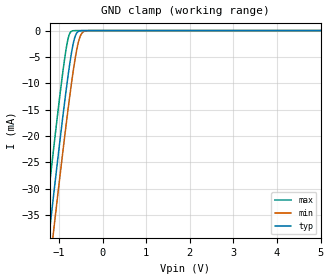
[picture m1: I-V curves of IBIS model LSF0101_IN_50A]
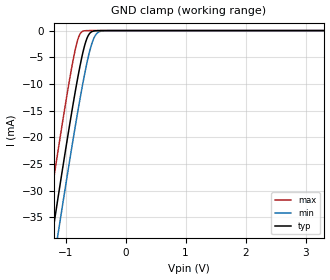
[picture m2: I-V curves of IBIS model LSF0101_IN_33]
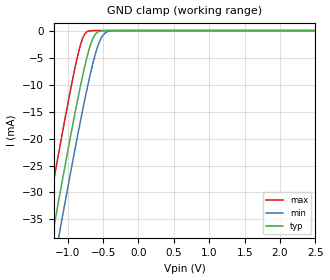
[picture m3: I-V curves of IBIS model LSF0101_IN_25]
|Texas Instruments Incorporated
| Single Bidirectional Multi-Voltage Level Translator
| for Open-Drain & Push-Pull Application
| Marketing part#   Digital Voltage Range   Package-type   #pins
| LSF0102DCT   1.2V-5.5V   SSOP   8
| LSF0102DCU   1.2V-5.5V   VSSOP   8
| This device can be powered at the following Vccs:
|  5 volt Vcc
|  3.3 volt Vcc
|  2.5 volt Vcc
|  1.8 volt Vcc
|  1.2 volt Vcc
[IBIS Ver]   4.1
[File name]   lsf0102.ibs
[File Rev]   1.0
[Date]   08/01/2014
[Source]
| Texas Instruments Incorporated.
| 12500 TI Blvd
| Dallas, TX -75243
[Notes]   Revision History:
| Rev 1.0: 8/01/2014
| - Initial version of the model
| - Model generated from simulations in TISPICE
| - C_comp although listed in numerical order of value are
|   obtained from varying PVT conditions. For PVT conditions for
|   each specific value refer the buffer description under
|   respective [Model]. IBIS model user is responsible for using
|   appropriate C_comp to simulate for Signal Integrity.
| - Non-monotonic data due to FET characteristics.
| - POWER clamp data deleted as there is no power-clmp diode.
[Disclaimer]
| This model is designed as an aid for customers of Texas Instruments.
| TI and its licensors and suppliers make no warranties, either expressed
| or implied, with respect to this  model, including the warranties of
| merchantability or fitness for a particular purpose. The model is
| provided solely on an "as is" basis. The entire risk as to its quality
| and performance is with the customer.
| This file provides unique models under the [Model Selector] for each Vcc.
| For operation at a specific Vcc, select the appropriate model after each
| [Model Selector] keyword.
[Copyright]
 (C) Copyright 2014 Texas Instruments Incorporated.All rights reserved.
|   Device
[Component]   LSF0102DCT
[Manufacturer]   TI
[Package]   |SSOP, 8 pin DCT
|   typ   min   max
R_pkg   0.0495   0.0439   0.0557
L_pkg   2.0203n   1.8892n   2.1572n
C_pkg   0.0923p   0.0784p   0.1044p
[Pin]  signal_name   model_name   R_pin   L_pin   C_pin
1   GND   GND   0.05353   2.1389n   0.1044p
2   VREF_A   LSF0101_IO   0.04507   1.9025n   0.0813p
3   A1   LSF0101_IO   0.04637   1.9443n   0.0839p
4   A2   LSF0101_IO   0.05217   2.0711n   0.1026p
5   B2   LSF0101_IO   0.05569   2.1572n   0.1042p
6   B1   LSF0101_IO   0.04687   1.9375n   0.0793p
7   VREF_B   LSF0101_IO   0.04389   1.8892n   0.0784p
8   EN   LSF0101_IN   0.05272   2.1213n   0.1042p
[Series Switch Groups]
| Function Group States
On  1 /   | A1 -> B1 EN HIGH
Off 1 /   | EN LOW
[Series Pin Mapping]   pin_2   model_name   function_table_group
3   6   LSF0101_IO_S   1
4   5   LSF0101_IO_S   1
|   Device
[Component]   LSF0102DCU
[Manufacturer]   TI
[Package]   |VSSOP, 8 pin DCU
|   typ   min   max
R_pkg   0.0422   0.0373   0.0480
L_pkg   0.9667n   0.8401n   1.1004n
C_pkg   0.0504p   0.0475p   0.0527p
[Pin]  signal_name   model_name   R_pin   L_pin   C_pin
1   GND   GND   0.04804   1.1004n   0.0494p
2   VREF_A   LSF0101_IO   0.03770   0.8401n   0.0524p
3   A1   LSF0101_IO   0.03799   0.8707n   0.0527p
4   A2   LSF0101_IO   0.04650   1.0833n   0.0489p
5   B2   LSF0101_IO   0.04545   1.0350n   0.0475p
6   B1   LSF0101_IO   0.03792   0.8603n   0.0525p
7   VREF_B   LSF0101_IO   0.03729   0.8532n   0.0520p
8   EN   LSF0101_IN   0.04638   1.0906n   0.0476p
[Series Switch Groups]
| Function Group States
On  1 /   | A1 -> B1 EN HIGH
Off 1 /   | EN LOW
[Series Pin Mapping]   pin_2   model_name   function_table_group
3   6   LSF0101_IO_S   1
4   5   LSF0101_IO_S   1
| Model LSF0101_IN
[Model Selector]   LSF0101_IN
LSF0101_IN_50A   5 volt Vcc
LSF0101_IN_33   3.3 volt Vcc
LSF0101_IN_25   2.5 volt Vcc
LSF0101_IN_18   1.8 volt Vcc
LSF0101_IN_12A   1.2 volt Vcc
| Model LSF0101_IO
[Model Selector]   LSF0101_IO
LSF0101_IO_50A   5 volt Vcc
LSF0101_IO_33   3.3 volt Vcc
LSF0101_IO_25   2.5 volt Vcc
LSF0101_IO_18   1.8 volt Vcc
LSF0101_IO_12A   1.2 volt Vcc
| Model LSF0101_IO_S
[Model Selector]   LSF0101_IO_S
LSF0101_IO_50A_S   5 volt Vcc
LSF0101_IO_33_S   3.3 volt Vcc
LSF0101_IO_25_S   2.5 volt Vcc
LSF0101_IO_18_S   1.8 volt Vcc
LSF0101_IO_12A_S   1.2 volt Vcc
[Model]   LSF0101_IO_50A_S
Model_type  Series_switch
| variable   typ   min   max
C_comp   0   0   0
[Temperature Range]   40   100   -40
| Ambient temperature   25   85   -40
[Voltage range]   5   5   5
[On]
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[Off]
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[Model]   LSF0101_IO_33_S
Model_type  Series_switch
| variable   typ   min   max
C_comp   0   0   0
[Temperature Range]   40   100   -40
| Ambient temperature   25   85   -40
[Voltage range]   3.3   3   3.6
[On]
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[Off]
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[Model]   LSF0101_IO_25_S
Model_type  Series_switch
| variable   typ   min   max
C_comp   0   0   0
[Temperature Range]   40   100   -40
| Ambient temperature   25   85   -40
[Voltage range]   2.5   2.3   2.7
[On]
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[Off]
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[Model]   LSF0101_IO_18_S
Model_type  Series_switch
| variable   typ   min   max
C_comp   0   0   0
[Temperature Range]   40   100   -40
| Ambient temperature   25   85   -40
[Voltage range]   1.8   1.65   1.95
[On]
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[Off]
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[Model]   LSF0101_IO_12A_S
Model_type  Series_switch
| variable   typ   min   max
C_comp   0   0   0
[Temperature Range]   40   100   -40
| Ambient temperature   25   85   -40
[Voltage range]   1.2   1.2   1.2
[On]
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[Off]
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| Models and submodels in the file (15): LSF0101_IN_50A (Input), LSF0101_IN_33 (Input), LSF0101_IN_25 (Input), LSF0101_IN_18 (Input), LSF0101_IN_12A (Input), LSF0101_IO_50A_S (Series_switch), LSF0101_IO_50A (Terminator), LSF0101_IO_33_S (Series_switch), LSF0101_IO_33 (Terminator), LSF0101_IO_25_S (Series_switch), LSF0101_IO_25 (Terminator), LSF0101_IO_18_S (Series_switch), LSF0101_IO_18 (Terminator), LSF0101_IO_12A_S (Series_switch), LSF0101_IO_12A (Terminator)
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[Model]   LSF0101_IN_50A
Model_type  Input
Vinl=0.6
Vinh=5
| variable   typ   min   max
C_comp   6.26pF   4.66pF   9.23pF
[Temperature Range]   40   100   -40
| Ambient temperature   25   85   -40
[Voltage range]   5   5   5
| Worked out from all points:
|   GND clamp passes 1 mA (typ) near -0.62 V on its own axis
[GND Clamp]
| PCA9306_IN_50A
|   Voltage   I(typ)   I(min)   I(max)
-5V       -328.9mA   -335.1mA   -321mA
-1.365V   -49.02mA   -55.82mA   -40.25mA
-1.325V   -46.04mA   -52.85mA   -37.26mA
-1.215V   -37.92mA   -44.74mA   -29.12mA
-1.12V    -30.99mA   -37.81mA   -22.19mA
-850mV    -12.22mA   -18.79mA   -4.2mA
-780mV    -7.858mA   -14.16mA   -1.166mA
-710mV    -4.062mA   -9.799mA   -118uA
-635mV    -1.238mA   -5.618mA   -5.709uA
-555mV    -167.5uA   -2.206mA   -200.7nA
-405mV    -1.746uA   -97.01uA   -397.3pA
5V        97.63pA    2.873nA    90.01pA
[Model]   LSF0101_IN_33
Model_type  Input
Vinl=0.6
Vinh=3.6
| variable   typ   min   max
C_comp   6.06pF   4.74pF   7.90pF
[Temperature Range]   40   100   -40
| Ambient temperature   25   85   -40
[Voltage range]   3.3   3   3.6
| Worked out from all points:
|   GND clamp passes 1 mA (typ) near -0.62 V on its own axis
[GND Clamp]
| PCA9306_IN_33
|   Voltage   I(typ)   I(min)   I(max)
-3.3V     -197mA     -203.5mA   -188.9mA
-1.36V    -48.65mA   -55.45mA   -39.88mA
-1.315V   -45.3mA    -52.12mA   -36.52mA
-1.23V    -39.02mA   -45.85mA   -30.22mA
-1.19V    -36.09mA   -42.91mA   -27.28mA
-1.115V   -30.63mA   -37.45mA   -21.83mA
-850mV    -12.22mA   -18.79mA   -4.2mA
-715mV    -4.305mA   -10.1mA    -142.6uA
-635mV    -1.238mA   -5.618mA   -5.709uA
-555mV    -167.5uA   -2.206mA   -200.7nA
-405mV    -1.746uA   -97.01uA   -397.3pA
3.3V      64.05pA    2.84nA     56.56pA
[Model]   LSF0101_IN_25
Model_type  Input
Vinl=0.6
Vinh=2.7
| variable   typ   min   max
C_comp   5.97pF   4.76pF   7.97pF
[Temperature Range]   40   100   -40
| Ambient temperature   25   85   -40
[Voltage range]   2.5   2.3   2.7
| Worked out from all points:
|   GND clamp passes 1 mA (typ) near -0.62 V on its own axis
[GND Clamp]
| PCA9306_IN_25
|   Voltage   I(typ)   I(min)   I(max)
-2.5V     -135.3mA   -141.9mA   -127mA
-1.335V   -46.79mA   -53.6mA    -38.01mA
-1.22V    -38.29mA   -45.11mA   -29.48mA
-1.185V   -35.72mA   -42.55mA   -26.92mA
-1.12V    -30.99mA   -37.81mA   -22.19mA
-855mV    -12.54mA   -19.12mA   -4.472mA
-785mV    -8.155mA   -14.49mA   -1.319mA
-720mV    -4.553mA   -10.4mA    -171.8uA
-640mV    -1.37mA    -5.873mA   -7.034uA
-560mV    -192.8uA   -2.373mA   -247.3nA
-415mV    -2.384uA   -124.1uA   -599.6pA
2.5V      48.96pA    2.825nA    41.29pA
